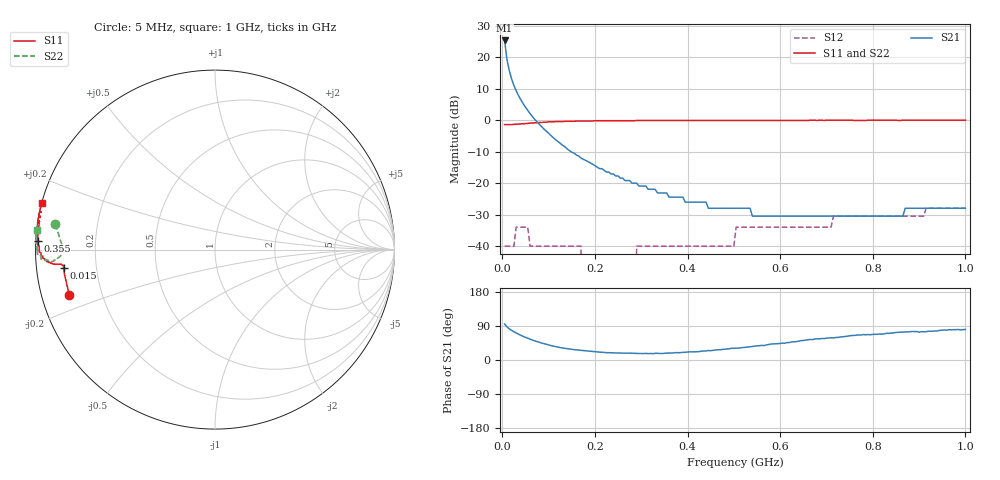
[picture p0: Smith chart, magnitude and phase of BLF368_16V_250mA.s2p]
! Filename:  BLF368_16V_250mA.s2p
! Philips part #: BLF368  !date: 21-05-2003
!16V @250 mA
!D:\Vee measurements\measurement data\VDMOST\BLF368\16V_250mA_#1
# HZ S MA R 50
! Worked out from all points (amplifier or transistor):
!   200 points, 5 MHz to 1 GHz, reference 50 ohm
!   highest |S21| = 25.3 dB at 5 MHz (marker M1)
!   |S21| within 3 dB of that: start of sweep to 7.529 MHz
!   S11 on the Smith chart (normalised r, x): 5 MHz: 0.08, -0.15; 15 MHz: 0.08, -0.06; 355 MHz: 0.01, +0.02; 1 GHz: -0.00, +0.13
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5000000  0.85 -162.7  18.43 94.9  0.01 3.0  0.9 170.9
1e7  0.85 -170.6  9.31 87.3  0.01 21.8  0.87 175.3
1.5e7  0.85 -173.1  6.16 82.3  0.01 22.2  0.86 177.1
2e7  0.85 -174.1  4.54 78.2  0.01 18.4  0.85 178.5
2.5e7  0.86 -174.4  3.58 74.8  0.01 13.4  0.86 179.5
3e7  0.86 -174.6  2.94 71.3  0.02 8.2  0.86 -179.9
4e7  0.87 -174.6  2.11 65.2  0.02 -0.4  0.86 -178.4
5.5e7  0.89 -174.7  1.43 57.3  0.02 -10.6  0.88 -176.8
6e7  0.9 -174.8  1.27 54.9  0.01 -13.4  0.88 -176.5
9.5e7  0.93 -175.8  0.67 41.3  0.01 -26.3  0.92 -175.8
1.7e8  0.97 -178.3  0.25 25.4  0.01 -22.9  0.97 -176.8
1.75e8  0.97 -178.5  0.24 24.8  0 -20.6  0.97 -176.9
2.85e8  0.98 178.7  0.1 17.6  0 67.7  0.99 -178.9
2.9e8  0.99 178.5  0.1 17.5  0.01 69.3  0.99 -178.9
3.4e8  0.99 177.4  0.07 17.2  0.01 76.4  0.99 -179.6
3.55e8  0.99 177.2  0.07 18.2  0.01 78.1  0.99 -179.8
5e8  0.99 174.3  0.04 30.7  0.01 88.3  1 178.5
5.05e8  0.99 174.3  0.04 31.4  0.02 88.3  1 178.5
6.7e8  1 171.3  0.03 54.0  0.02 90.5  1 176.8
7.15e8  1 170.5  0.03 58.2  0.03 90.6  1 176.5
8.35e8  1 168.3  0.03 70.2  0.03 92.8  1 175.4
1e9  1 165.1  0.04 80.6  0.04 91.7  1 173.6
